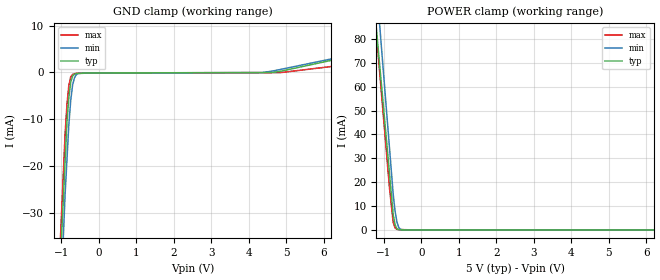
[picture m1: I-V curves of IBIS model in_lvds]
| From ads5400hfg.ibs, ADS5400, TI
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[Model] in_lvds
Model_type Input
Vinl = 900.000mV
Vinh = 1.60000V
C_comp 433.000fF 428.000fF 444.000fF
| variable typ   min   max
[Voltage Range] 5.00000V 4.75000V 5.25000V
[POWER Clamp Reference] 5.00000V 4.75000V 5.25000V
[GND Clamp Reference] 0.00000V 0.00000V 0.00000V
[Temperature Range] 25   85   -40
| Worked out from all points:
|   GND clamp passes 1 mA (typ) near -0.71 V on its own axis
|   POWER clamp passes 1 mA (typ) near -0.66 V on its own axis
[GND Clamp]
-5V       -715.8mA   -824.3mA   -749.8mA
-900mV    -19.16mA   -26.17mA   -13.33mA
-850mV    -10.67mA   -18.71mA   -6.945mA
-800mV    -5.369mA   -11.26mA   -2.813mA
-750mV    -2.124mA   -6.043mA   -960.1uA
-700mV    -780.9uA   -2.709mA   -429.8uA
-650mV    -383.5uA   -1.164mA   -299.5uA
-600mV    -219.8uA   -484.7uA   -169.2uA
-275mV    -109.8uA   -109.5uA   -110uA
4.35V     -40.33uA   -34.37uA   -45.59uA
4.6V      -36.58uA   257uA      -42.11uA
10V       9.109mA    9.178mA    4.915mA
[POWER Clamp]
-5V       743.8mA    849.8mA    785mA
-1.05V    58.47mA    73.87mA    54.76mA
-850mV    23.77mA    34.58mA    17.79mA
-750mV    6.416mA    14.94mA    3.193mA
-700mV    2.211mA    7.835mA    815.7uA
-650mV    484.4uA    3.302mA    288.3uA
-600mV    67.25uA    1.004mA    180.4uA
-550mV    56.04uA    213.5uA    159.2uA
-450mV    33.62uA    19uA       116.7uA
10V       0A         0A         0A
